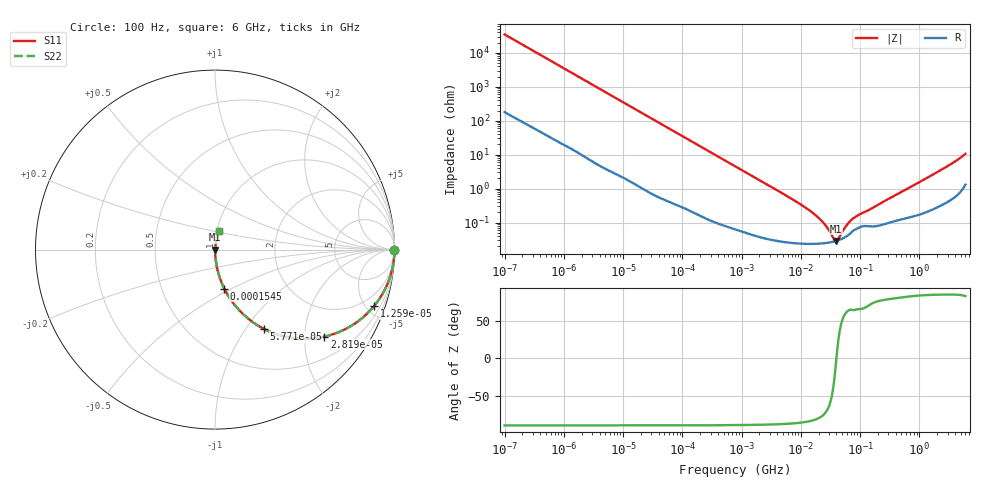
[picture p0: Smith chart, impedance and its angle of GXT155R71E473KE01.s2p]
!Murata Part Number: GXT155R71E473KE01
!These Parameters are Measured in Series Mode Connection
!Data Generated on Jan 08, 2026
!  o--ll--o
!Port1  Port2
!  o------o
!Operation Temp=25[degC], DC Bias Voltage=0[V]
!Freq. Start=100[Hz] Stop=6[GHz] 401[Steps]
# Hz S RI R 50
!Freq.(Hz) S11(Real) S11(Imag) S21(Real) S21(Imag) S12(Real) S12(Imag) S22(Real) S22(Imag)
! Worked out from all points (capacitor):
!   401 points, 100 Hz to 6 GHz, reference 50 ohm
!   read as one part in series: C = 46 nF near 109 Hz
!   lowest |Z| = 29.1 mohm at 39.84 MHz (marker M1)
!   series resonance near 39.92 MHz, so ESL is about 350 pH
!   S11 on the Smith chart (normalised r, x): 100 Hz: open; 12.59 kHz: 1.03, -5.59; 28.19 kHz: 1.02, -2.50; 57.71 kHz: 1.01, -1.23; 154.5 kHz: 1.00, -0.46; 6 GHz: 1.03, +0.21
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100  1 -0.00289  2.33e-05 0.00289  2.33e-05 0.00289  1 -0.00289
2008  0.9964 -0.0572  0.00361 0.0572  0.00361 0.0572  0.9964 -0.0572
5378  0.9762 -0.1497  0.0238 0.1497  0.0238 0.1497  0.9762 -0.1497
12592  0.8849 -0.3162  0.1151 0.3162  0.1151 0.3162  0.8849 -0.3162
28191  0.6095 -0.4848  0.3905 0.4848  0.3905 0.4848  0.6095 -0.4848
40335  0.4343 -0.4925  0.5657 0.4925  0.5657 0.4925  0.4343 -0.4925
57709  0.2743 -0.4427  0.7257 0.4427  0.7257 0.4427  0.2743 -0.4427
90302  0.1353 -0.3382  0.8647 0.3382  0.8647 0.3382  0.1353 -0.3382
154540  0.0519 -0.2175  0.9481 0.2175  0.9481 0.2175  0.0519 -0.2175
316350  0.0136 -0.111  0.9864 0.111  0.9864 0.111  0.0136 -0.111
774597  0.00276 -0.0461  0.9972 0.0461  0.9972 0.0461  0.00276 -0.0461
6353432  0.000288 -0.00556  0.9997 0.00556  0.9997 0.00556  0.000288 -0.00556
1.555665e7  0.000241 -0.00198  0.9998 0.00198  0.9998 0.00198  0.000241 -0.00198
2.327686e7  0.000246 -0.00103  0.9998 0.00103  0.9998 0.00103  0.000246 -0.00103
3.64232e7  0.000279 -0.000167  0.9997 0.000167  0.9997 0.000167  0.000279 -0.000167
3.983537e7  0.000291 -3.8e-06  0.9997 3.8e-06  0.9997 3.8e-06  0.000291 -3.8e-06
4.35672e7  0.000306 0.000159  0.9997 -0.000159  0.9997 -0.000159  0.000306 0.000159
5.960426e7  0.0004 0.000745  0.9996 -0.000745  0.9996 -0.000745  0.0004 0.000745
7.455971e7  0.00056 0.00116  0.9994 -0.00116  0.9994 -0.00116  0.00056 0.00116
3.124326e8  0.00102 0.00508  0.999 -0.00508  0.999 -0.00508  0.00102 0.00508
2.450438e9  0.0047 0.037  0.9953 -0.037  0.9953 -0.037  0.0047 0.037
6e9  0.0236 0.1016  0.9764 -0.1016  0.9764 -0.1016  0.0236 0.1016
